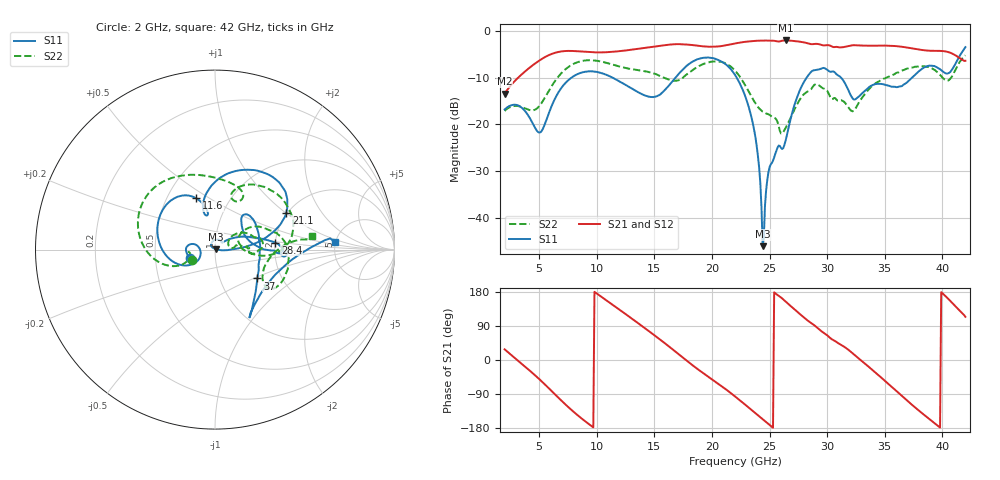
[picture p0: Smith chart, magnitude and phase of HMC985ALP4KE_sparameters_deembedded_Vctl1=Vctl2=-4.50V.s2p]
!s2p File: Measurements: S11, S21, S12, S22
# GHz S dB R 50.0
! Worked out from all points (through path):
!   401 points, 2 GHz to 42 GHz, reference 50 ohm
!   highest |S21| = -2.06 dB at 26.4 GHz (marker M1); lowest = -13.4 dB at 2 GHz (marker M2)
!   lowest |S11| = -46.1 dB at 24.4 GHz (marker M3), VSWR 1.01, Z = 50.5 + j0.199 ohm
!   |S11| at or under -10 dB: start of sweep to 7.82 GHz; 22.14 GHz to 28.22 GHz (6.083 GHz wide, 24.2 % of centre); 31.2 GHz to 37.38 GHz (6.187 GHz wide, 18 % of centre)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
!   |S22| runs from -22.0 to -5.2 dB; largest |S21 - S12| = 0.00074
!   S11 on the Smith chart (normalised r, x): 2 GHz: 0.76, -0.07; 11.6 GHz: 0.70, +0.44; 21.1 GHz: 1.97, +1.01; 28.4 GHz: 2.01, +0.17; 37 GHz: 1.51, -0.53; 42 GHz: 4.93, +0.74
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2  -16.83 -161.8  -13.44 28.2  -13.44 28.2  -17.14 -155.6
5  -21.77 -173.2  -6.38 -50.2  -6.38 -50.2  -16.13 -160.1
6.3  -14.87 -150.6  -4.76 -88.4  -4.77 -88.4  -11.01 -161.9
8.7  -8.93 150.2  -4.44 -154.7  -4.44 -154.7  -6.46 151.1
11.6  -10.32 110.2  -4.45 140.8  -4.45 140.8  -7.38 103.2
13.6  -13.15 101.3  -3.85 96.9  -3.85 96.9  -8.42 75.4
15.4  -13.78 106.2  -3.25 56.1  -3.25 56.1  -9.54 62.0
17.9  -7.29 80.0  -2.95 -4.0  -2.95 -4.0  -9.16 72.0
21.1  -6.99 27.3  -3.15 -74.8  -3.15 -74.8  -6.89 15.7
22  -9.41 16.8  -2.71 -96.0  -2.71 -96.0  -8.51 0.3
23.6  -20.44 0.5  -2.18 -135.8  -2.18 -135.8  -14.82 -4.2
24  -27.02 -5.2  -2.12 -145.8  -2.11 -145.8  -16.32 1.5
24.4  -46.09 23.4  -2.09 -155.9  -2.09 -155.9  -17.30 7.5
25.1  -28.61 124.6  -2.12 -173.7  -2.12 -173.7  -18.16 11.0
26.4  -23.44 41.6  -2.06 154.1  -2.06 154.1  -20.79 33.2
28.4  -9.39 6.5  -2.73 102.0  -2.73 102.0  -12.87 17.9
28.7  -8.58 1.5  -2.86 95.8  -2.87 95.8  -12.17 16.1
32.5  -14.56 32.8  -3.10 10.0  -3.10 10.0  -16.46 28.3
35.4  -11.79 18.6  -3.18 -65.5  -3.18 -65.5  -9.76 19.1
37  -10.88 -34.2  -3.60 -108.6  -3.60 -108.6  -8.06 4.6
39.8  -8.22 -57.0  -4.30 -178.4  -4.30 -178.3  -9.42 -35.5
42  -3.49 3.5  -6.42 114.0  -6.43 114.0  -5.24 8.1
